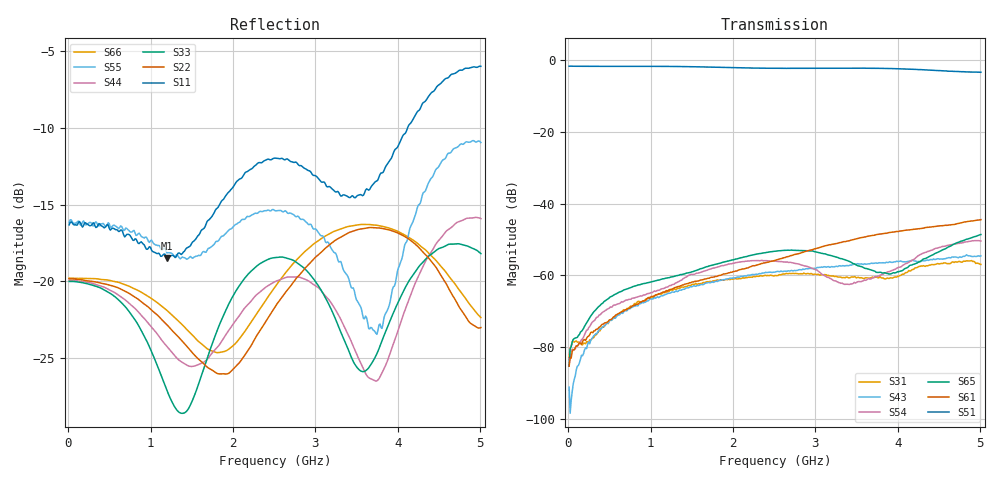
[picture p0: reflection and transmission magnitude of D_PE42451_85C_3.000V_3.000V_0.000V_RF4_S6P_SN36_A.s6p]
! Device ID: PE42451
! Serial: 36
! Insertion: A
! Temp: 85C
! VDD: 3.000
! Control_Hi: 100.000
! Control_Lo: 0.000
! Logic State: RF4
! Port 1: RFC
! Port 2: RF1
! Port 3: RF2
! Port 4: RF3
! Port 5: RF4
! Port 6: RF5
! V1 = 0.00
! V2 = 0.00
! V3 = 3.00
! V4 = 0.00
! IDD: 1.383520e-05
#  Hz  S  RI  R  50
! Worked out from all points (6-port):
!   401 points, 10 MHz to 5.01 GHz, reference 50 ohm
!   strongest paths, dB at 10 MHz, 1.26 GHz, 2.51 GHz, 3.76 GHz, 5.01 GHz:
!     S51: -1.6, -1.7, -2.2, -2.2, -3.3
!     S61: -85.3, -63.8, -55.8, -48.6, -44.5
!     S65: -85.3, -60.4, -53.3, -59.2, -48.6
!     S54: -83.4, -62.6, -56.0, -60.3, -50.4
!     S43: -91.2, -64.6, -59.1, -56.6, -54.5
!     S31: -82.9, -64.1, -60.0, -60.7, -56.9
!   lowest |S11| = -18.5 dB at 1.198 GHz (marker M1), VSWR 1.27, Z = 56.4 - j11 ohm
!   |S11| at or under -10 dB: start of sweep to 4.12 GHz
